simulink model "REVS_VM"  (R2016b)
settings: Solver=ode3  StartTime=REVS.sim_start_time_secs  StopTime=Inf  FixedStep=REVS.sim_step_time_secs  MaxStep=REVS.sim_step_time_secs  EnableMultiTasking=on
StopFcn:
  | postproc_datalog;
  | postproc_audit;
  | postproc_result;
model workspace (MATLAB code in the model file):
  other statements: REVS_setup_variants
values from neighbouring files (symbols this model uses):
  accessory = class_accessory_data    [class_test_data.m]
  battery = class_battery_data    [class_accessory_data.m]    (also in class_REVS_electric.m = class_REVS_battery)
  brake = struct(	'max_torque_Nm',[], 						'proportion_norm',1.0, 						'inertia_kgm2',0.0)    [class_REVS_drive_axle.m]
  engine = class_engine_data    [class_test_data.m]
  final_drive = struct(	'gear_ratio',[], 								'efficiency_norm',[], 								'inertia_kgm2',[] )    [class_REVS_drive_axle.m]
  gear = class_REVS_gearbox    [class_REVS_AT_transmission.m]
  tire = struct(	'radius_m',[], 						'rolling_resistance_coefficient',0, 						'vehicle_weight_norm',1.0,  						'wheel_slip_torque_Nm',[],  						'inertia_kgm2',0.0)    [class_REVS_drive_axle.m]
  torque_converter = class_REVS_torque_converter    [class_REVS_AT_transmission.m]
  transmission = class_transmission_data    [class_test_data.m]
  vehicle = class_vehicle_data    [class_test_data.m]
undefined symbols (not defined in the file or in its folder): alternator, ambient, controls, convert, DelayTimeSecs, drive_cycle, driver, electric, gear_strategy, InitialCondition, InitialValue, LoadSource, LookupStructure, MultiplyPosInputs, Normalize, NumPhases, REVS, SpeedSource, starter, tableshift, UpperSaturationLimit, Value, VerboseLevel, VerboseSignal
libraries: simulink x153
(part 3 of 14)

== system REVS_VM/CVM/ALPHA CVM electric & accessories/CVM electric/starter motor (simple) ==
  system_bus : Inport
  batt_volts_V : Inport  Port=2
  spd_in_radps : Inport  Port=3
  Bus Selector : BusSelector  OutputSignals=powertrain.control.ctrl_eng_on,powertrain.engine.ISC_state
  Divide1 : Product  Inputs=**//
  Divide2 : Product  Inputs=*/*
  Input Output Elec Mech E&P Nm radps V A : Subsystem
  PID Controller : simulink/Continuous/PID Controller  Controller=PID  TimeDomain=Continuous-time  SampleTime=-1  IntegratorMethod=Forward Euler  FilterMethod=Forward Euler  Form=Parallel  UseFilter=on  ControllerParametersSource=internal  P=10  I=10  D=0  N=1  InitialConditionSource=internal  InitialConditionForIntegrator=0  InitialConditionForFilter=0  ExternalReset=rising  ZeroCross=off  LimitOutput=on  UpperSaturationLimit=starter.max_torque_Nm  LowerSaturationLimit=0  LinearizeAsGain=on  AntiWindupMode=none  Kb=1  TrackingMode=off  Kt=1  PParamMin=[]  PParamMax=[]  IParamMin=[]  IParamMax=[]  DParamMin=[]  DParamMax=[]  NParamMin=[]  NParamMax=[]  KbParamMin=[]  KbParamMax=[]  KtParamMin=[]  KtParamMax=[]  POutMin=[]  POutMax=[]  IOutMin=[]  IOutMax=[]  DOutMin=[]  DOutMax=[]  NOutMin=[]  NOutMax=[]  KbOutMin=[]  KbOutMax=[]  KtOutMin=[]  KtOutMax=[]  IntegratorOutMin=[]  IntegratorOutMax=[]  FilterOutMin=[]  FilterOutMax=[]  SumOutMin=[]  SumOutMax=[]  SumI1OutMin=[]  SumI1OutMax=[]  SumI2OutMin=[]  SumI2OutMax=[]  SumI3OutMin=[]  SumI3OutMax=[]  SumDOutMin=[]  SumDOutMax=[]  SaturationOutMin=[]  SaturationOutMax=[]  IntegratorContinuousStateAttributes=''  IntegratorStateMustResolveToSignalObject=off  IntegratorRTWStateStorageClass=Auto  FilterContinuousStateAttributes=''  FilterStateMustResolveToSignalObject=off  FilterRTWStateStorageClass=Auto  DifferentiatorICPrevScaledInput=0  DifferentiatorOutMin=[]  DifferentiatorOutMax=[]
  Product : Product
  Rate Limiter : RateLimiter  RisingSlewLimit=electric.starter.max_torque_Nm * 10  FallingSlewLimit=-Inf
  Saturation1 : Saturate  UpperLimit=Inf  LowerLimit=eps
  Sum2 : Sum  Inputs=+-|
  cranking_speed_radps : Constant  Value=starter.cranking_speed_radps
  efficiency_norm : Constant  Value=starter.efficiency_norm
  efficiency_norm1 : Constant  Value=starter.rated_voltage_V
  inertia kgm2 : Constant  Value=starter.inertia_kgm2
  starter control : Subsystem
  to datalog1 : Subsystem
  to datalog2 : Subsystem
  to datalog3 : Subsystem
  trq_out_Nm : Outport
  iner_out_kgm2 : Outport  Port=2
  curr_out_A : Outport  Port=3
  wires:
  efficiency_norm1/1 -> Divide2/2
  Product/1 -> Divide2/1
  Divide1/1 -> Input Output Elec Mech E&P Nm radps V A/2(curr_in_A), curr_out_A/1
  Bus Selector/1 -> starter control/1(eng_on)  "<ctrl_eng_on>"
  system_bus/1 -> Bus Selector/1
  starter control/1(state) -> PID Controller/2, to datalog2/1(Var), Product/2
  PID Controller/1 -> Product/1, to datalog1/1(Var)
  Sum2/1 -> PID Controller/1
  cranking_speed_radps/1 -> Sum2/1
  Saturation1/1 -> Divide1/4
  efficiency_norm/1 -> Divide1/3
  batt_volts_V/1 -> Divide2/3, Input Output Elec Mech E&P Nm radps V A/1(volts_in_V), Saturation1/1, starter control/2(batt_volts_V)
  spd_in_radps/1 -> starter control/3(spd_in_radps), Sum2/2, Input Output Elec Mech E&P Nm radps V A/4(spd_out_radps), Divide1/2
  Divide2/1 -> to datalog3/1(Var), Rate Limiter/1
  inertia kgm2/1 -> iner_out_kgm2/1, Input Output Elec Mech E&P Nm radps V A/5(iner_out_kgm2)
  Rate Limiter/1 -> Input Output Elec Mech E&P Nm radps V A/3(trq_out_Nm), Divide1/1, trq_out_Nm/1
  Bus Selector/2 -> starter control/4(ISC_state)  "<ISC_state>"

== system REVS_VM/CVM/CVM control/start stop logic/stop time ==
  bool : Inport
  Constant : Constant  Value=Normalize
  Data Type Conversion2 : DataTypeConversion  OutDataTypeStr=double
  Integrator1 : Integrator  ExternalReset=falling  LimitOutput=on  UpperSaturationLimit=UpperSaturationLimit  LowerSaturationLimit=0
  Switch : Switch  Criteria=u2 > Threshold
  normalize : Gain  Gain=1/UpperSaturationLimit
  out : Outport
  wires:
  Switch/1 -> out/1
  normalize/1 -> Switch/1
  Integrator1/1 -> Switch/3, normalize/1
  Constant/1 -> Switch/2
  bool/1 -> Data Type Conversion2/1
  Data Type Conversion2/1 -> Integrator1/1, Integrator1/2

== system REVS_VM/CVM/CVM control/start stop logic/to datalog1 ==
  Var : Inport
  Constant : Constant  Value=VerboseSignal
  Constant1 : Constant  Value=VerboseLevel
  Relational Operator : RelationalOperator  OutDataTypeStr=boolean  ZeroCross=off
  Subsystem : Subsystem
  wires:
  Constant1/1 -> Relational Operator/2
  Constant/1 -> Relational Operator/1
  Relational Operator/1 -> Subsystem/Enable
  Var/1 -> Subsystem/1(In1)

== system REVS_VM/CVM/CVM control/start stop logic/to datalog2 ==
  Var : Inport
  Constant : Constant  Value=VerboseSignal
  Constant1 : Constant  Value=VerboseLevel
  Relational Operator : RelationalOperator  OutDataTypeStr=boolean  ZeroCross=off
  Subsystem : Subsystem
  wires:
  Constant1/1 -> Relational Operator/2
  Constant/1 -> Relational Operator/1
  Relational Operator/1 -> Subsystem/Enable
  Var/1 -> Subsystem/1(In1)

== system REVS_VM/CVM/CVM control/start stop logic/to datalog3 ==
  Var : Inport
  Constant : Constant  Value=VerboseSignal
  Constant1 : Constant  Value=VerboseLevel
  Relational Operator : RelationalOperator  OutDataTypeStr=boolean  ZeroCross=off
  Subsystem : Subsystem
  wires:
  Constant1/1 -> Relational Operator/2
  Constant/1 -> Relational Operator/1
  Relational Operator/1 -> Subsystem/Enable
  Var/1 -> Subsystem/1(In1)

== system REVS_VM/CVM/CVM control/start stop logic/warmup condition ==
  bus : Inport
  Bus Creator : BusCreator  Inputs=10
  Bus Creator1 : BusCreator  Inputs=2
  Bus Selector : BusSelector  OutputSignals=var_sigs.var_sig1  OutputAsBus=on
  Data Type Conversion : DataTypeConversion  OutDataTypeStr=double
  Display : Display
  Fcn : Fcn
  Variable {1..10} (10 alike) : Constant  Value=nan
  out : Outport
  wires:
  Data Type Conversion/1 -> Fcn/1
  Bus Selector/1 -> Data Type Conversion/1, Display/1
  Bus Creator1/1 -> Bus Selector/1
  Fcn/1 -> out/1
  bus/1 -> Bus Creator1/1  "system_bus"
  Bus Creator/1 -> Bus Creator1/2  "var_sigs"
  Variable 1/1 -> Bus Creator/1  "var_sig1"
  Variable 2/1 -> Bus Creator/2  "var_sig2"
  Variable 3/1 -> Bus Creator/3  "var_sig3"
  Variable 4/1 -> Bus Creator/4  "var_sig4"
  Variable 5/1 -> Bus Creator/5  "var_sig5"
  Variable 6/1 -> Bus Creator/6  "var_sig6"
  Variable 7/1 -> Bus Creator/7  "var_sig7"
  Variable 8/1 -> Bus Creator/8  "var_sig8"
  Variable 9/1 -> Bus Creator/9  "var_sig9"
  Variable 10/1 -> Bus Creator/10  "var_sig10"

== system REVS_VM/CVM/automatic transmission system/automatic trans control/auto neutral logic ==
  system_bus : Inport
  Bus Selector : BusSelector  OutputSignals=vehicle.veh_spd_mps,driver.accel_anticipate_bool,powertrain.control.ctrl_eng_on,powertrain.engine.eng_spd_radps
  Compare To Constant : simulink/Logic and Bit Operations/Compare To Constant  relop=>=  const=transmission.control.auto_neutral_delay_secs  OutDataTypeStr=boolean
  Compare To Zero4 : simulink/Logic and Bit Operations/Compare To Zero  relop=>  OutDataTypeStr=boolean
  Gain : Gain  Gain=1.5
  Logical Operator1 : Logic  Operator=OR  AllPortsSameDT=off  OutDataTypeStr=boolean
  Logical Operator2 : Logic  Inputs=4  AllPortsSameDT=off  OutDataTypeStr=boolean
  Logical Operator3 : Logic  Operator=NOT  AllPortsSameDT=off  OutDataTypeStr=boolean
  Logical Operator4 : Logic  Inputs=3  AllPortsSameDT=off  OutDataTypeStr=boolean
  Relational Operator : RelationalOperator  Operator=<  OutDataTypeStr=boolean
  auto neutral enable : Constant  Value=transmission.control.auto_neutral_enable
  crank speed : Constant  Value=electric.starter.cranking_speed_radps
  stop time : Subsystem
  stopped speed : simulink/Logic and Bit Operations/Compare To Constant  relop=<=  const=0.1  OutDataTypeStr=boolean
  to datalog1 : Subsystem
  warmup condition : Subsystem
  auto_neutral_bool : Outport
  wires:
  system_bus/1 -> warmup condition/1(bus), Bus Selector/1
  stop time/1(out) -> Compare To Constant/1
  stopped speed/1 -> stop time/1(bool), Logical Operator4/2
  warmup condition/1(out) -> Logical Operator2/4
  Compare To Zero4/1 -> Logical Operator3/1
  auto neutral enable/1 -> Logical Operator2/1
  Logical Operator3/1 -> Logical Operator2/3
  Bus Selector/1 -> stopped speed/1  "<veh_spd_mps>"
  Compare To Constant/1 -> Logical Operator2/2
  Logical Operator1/1 -> auto_neutral_bool/1, to datalog1/1(Var)
  Bus Selector/2 -> Compare To Zero4/1  "<accel_anticipate_bool>"
  Logical Operator4/1 -> Logical Operator1/2
  Logical Operator2/1 -> Logical Operator1/1
  Bus Selector/3 -> Logical Operator4/1  "<ctrl_eng_on>"
  Relational Operator/1 -> Logical Operator4/3
  Bus Selector/4 -> Relational Operator/1  "<eng_spd_radps>"
  crank speed/1 -> Gain/1
  Gain/1 -> Relational Operator/2

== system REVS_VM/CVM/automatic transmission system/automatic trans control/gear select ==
  note: 1) Only subsystems can be added as variant choices at this level 2) Blocks cannot be connected at this level as connectivity is automatically determined at simulation, based on the active variant
  system_bus : Inport
  ALPHAshift : Subsystem  VariantControl=get_REVS_transmission_gear_strategy_type(transmission) == enum_transmission_gear_select.ALPHAshift
  ALPHAshift_CVT : Subsystem  VariantControl=get_REVS_transmission_gear_strategy_type(transmission) == enum_transmission_gear_select.ALPHAshift_CVT
  SUBARUshift_CVT : Subsystem  VariantControl=get_REVS_transmission_gear_strategy_type(transmission) == enum_transmission_gear_select.subarushift_CVT
  autoshift 3 : Subsystem  VariantControl=get_REVS_transmission_gear_strategy_type(transmission) == enum_transmission_gear_select.autoshift3
  external gear select : Subsystem  VariantControl=get_REVS_transmission_gear_strategy_type(transmission) == enum_transmission_gear_select.externalshift
  external ratio select CVT : Subsystem  VariantControl=get_REVS_transmission_gear_strategy_type(transmission) == enum_transmission_gear_select.externalshift_CVT
  table gear select : Subsystem  VariantControl=get_REVS_transmission_gear_strategy_type(transmission) == enum_transmission_gear_select.tableshift
  table gear select with skip shift : Subsystem  VariantControl=get_REVS_transmission_gear_strategy_type(transmission) == enum_transmission_gear_select.tableshift_skipshift
  target_gear : Outport

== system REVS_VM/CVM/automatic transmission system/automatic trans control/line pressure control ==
  system_bus : Inport
  Rate Limiter : RateLimiter  RisingSlewLimit=transmission.control.line_press_rate_limit_barps  FallingSlewLimit=-Inf  InitialCondition=3
  dynamic lookup : Subsystem
  cmd_line_press_bar : Outport
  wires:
  system_bus/1 -> dynamic lookup/1(bus)
  dynamic lookup/1(out) -> Rate Limiter/1
  Rate Limiter/1 -> cmd_line_press_bar/1

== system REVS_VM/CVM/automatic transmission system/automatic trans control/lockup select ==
  note: 1) Only subsystems can be added as variant choices at this level 2) Blocks cannot be connected at this level as connectivity is automatically determined at simulation, based on the active variant
  gear_number : Inport
  system_bus : Inport  Port=2
  3-state lockup rules uber : Subsystem  VariantControl="get_REVS_transmission_tcc_strategy_type(transmission)  == enum_transmission_lockup_select.uber_dynamic_3state"
  "external lockup " : Subsystem  VariantControl="get_REVS_transmission_tcc_strategy_type(transmission)  == enum_transmission_lockup_select.external_lockup"
  lockup rules dynamic expression : Subsystem  VariantControl="get_REVS_transmission_tcc_strategy_type(transmission)  == enum_transmission_lockup_select.lockup_rules_dynamic_expression"
  lockup rules speed select : Subsystem  VariantControl="get_REVS_transmission_tcc_strategy_type(transmission)  == enum_transmission_lockup_select.lockup_rules_speed_select"
  lockup rules uber : Subsystem  VariantControl="get_REVS_transmission_tcc_strategy_type(transmission)  == enum_transmission_lockup_select.uber_dynamic"
  table lockup : Subsystem  VariantControl="get_REVS_transmission_tcc_strategy_type(transmission)  == enum_transmission_lockup_select.table_lockup"
  lockup_cmd : Outport

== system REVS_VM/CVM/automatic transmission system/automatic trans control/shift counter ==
  target_gear : Inport
  Constant : Constant  Value=transmission.gear.number
  Last Gear : Memory  X0=1
  Memory : Memory  X0=1
  Relational Operator : RelationalOperator  Operator===  OutDataTypeStr=boolean  ZeroCross=off
  Relational Operator1 : RelationalOperator  Operator=>  OutDataTypeStr=boolean  ZeroCross=off
  Relational Operator2 : RelationalOperator  Operator=<  OutDataTypeStr=boolean  ZeroCross=off
  Reshape : Reshape
  Switch : Switch  Criteria=u2 > Threshold
  downshifft result counter : Subsystem
  result integrator : Subsystem
  uppshift result counter : Subsystem
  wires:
  Relational Operator2/1 -> downshifft result counter/1(in)
  Last Gear/1 -> Relational Operator1/2, Relational Operator2/2
  Memory/1 -> Switch/3
  Switch/1 -> Memory/1, Relational Operator1/1, Relational Operator2/1, Last Gear/1
  target_gear/1 -> Switch/2, Switch/1, Relational Operator/1
  Reshape/1 -> Relational Operator/2
  Relational Operator/1 -> result integrator/1(in)
  Constant/1 -> Reshape/1
  Relational Operator1/1 -> uppshift result counter/1(in)

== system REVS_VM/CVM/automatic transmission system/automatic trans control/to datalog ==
  Var : Inport
  Constant : Constant  Value=VerboseSignal
  Constant1 : Constant  Value=VerboseLevel
  Relational Operator : RelationalOperator  OutDataTypeStr=boolean  ZeroCross=off
  Subsystem : Subsystem
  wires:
  Constant1/1 -> Relational Operator/2
  Constant/1 -> Relational Operator/1
  Relational Operator/1 -> Subsystem/Enable
  Var/1 -> Subsystem/1(In1)

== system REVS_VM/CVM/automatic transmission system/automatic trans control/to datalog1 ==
  Var : Inport
  Constant : Constant  Value=VerboseSignal
  Constant1 : Constant  Value=VerboseLevel
  Relational Operator : RelationalOperator  OutDataTypeStr=boolean  ZeroCross=off
  Subsystem : Subsystem
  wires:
  Constant1/1 -> Relational Operator/2
  Constant/1 -> Relational Operator/1
  Relational Operator/1 -> Subsystem/Enable
  Var/1 -> Subsystem/1(In1)

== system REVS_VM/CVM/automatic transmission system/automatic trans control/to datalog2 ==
  Var : Inport
  Constant : Constant  Value=VerboseSignal
  Constant1 : Constant  Value=VerboseLevel
  Relational Operator : RelationalOperator  OutDataTypeStr=boolean  ZeroCross=off
  Subsystem : Subsystem
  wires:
  Constant1/1 -> Relational Operator/2
  Constant/1 -> Relational Operator/1
  Relational Operator/1 -> Subsystem/Enable
  Var/1 -> Subsystem/1(In1)

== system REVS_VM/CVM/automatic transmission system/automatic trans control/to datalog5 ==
  Var : Inport
  Constant : Constant  Value=VerboseSignal
  Constant1 : Constant  Value=VerboseLevel
  Relational Operator : RelationalOperator  OutDataTypeStr=boolean  ZeroCross=off
  Subsystem : Subsystem
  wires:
  Constant1/1 -> Relational Operator/2
  Constant/1 -> Relational Operator/1
  Relational Operator/1 -> Subsystem/Enable
  Var/1 -> Subsystem/1(In1)

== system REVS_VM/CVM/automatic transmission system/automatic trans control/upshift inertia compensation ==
  system_bus : Inport
  Bus Selector : BusSelector  OutputSignals=powertrain.trans.ctrl.gear_num,powertrain.trans.core.gearbox.gb_curr_gear,powertrain.trans.ctrl.tcc_lockup_cmd_bool,powertrain.trans.trq_conv.tcc_lockup_bool
  Logical Operator : Logic  Operator=OR  AllPortsSameDT=off  OutDataTypeStr=boolean
  Logical Operator1 : Logic  AllPortsSameDT=off  OutDataTypeStr=boolean
  Relational Operator : RelationalOperator  Operator=>  OutDataTypeStr=boolean
  Relational Operator1 : RelationalOperator  Operator=>  OutDataTypeStr=boolean
  comp_iner_enable : Outport
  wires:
  Logical Operator1/1 -> Logical Operator/1
  Relational Operator/1 -> Logical Operator1/1
  system_bus/1 -> Bus Selector/1
  Relational Operator1/1 -> Logical Operator/2
  Bus Selector/4 -> Relational Operator1/2, Logical Operator1/2  "<tcc_lockup_bool>"
  Bus Selector/3 -> Relational Operator1/1  "<tcc_lockup_cmd_bool>"
  Logical Operator/1 -> comp_iner_enable/1  "eng_comp_iner_enable"
  Bus Selector/1 -> Relational Operator/1  "<gear_num>"
  Bus Selector/2 -> Relational Operator/2  "<gb_curr_gear>"

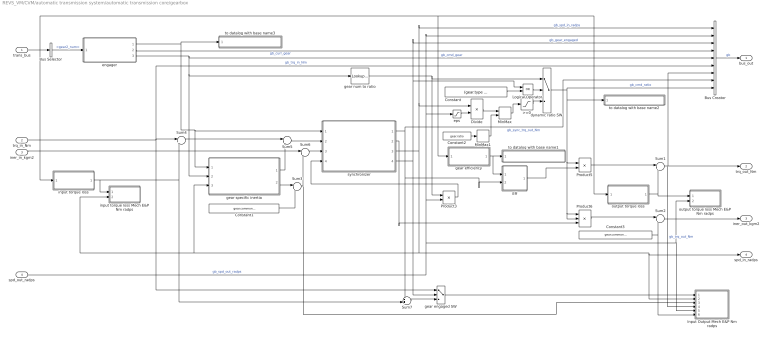
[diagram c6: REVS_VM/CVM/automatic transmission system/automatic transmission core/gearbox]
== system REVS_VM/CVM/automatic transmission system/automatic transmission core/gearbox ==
  trans_bus : Inport
  trq_in_Nm : Inport  Port=2
  iner_in_kgm2 : Inport  Port=3
  spd_out_radps : Inport  Port=4
  >=0 : Saturate  UpperLimit=Inf  LowerLimit=0
  Bus Creator : BusCreator  Inputs=9
  Bus Selector : BusSelector  OutputSignals=gear_num
  Constant : Constant  Value=(gear.type == enum_transmission_type.AMT) || (gear.type == enum_transmission_type.manual) || (gear.type == enum_transmission_type.DCT)
  Constant1 : Constant  Value=gear.common_input_inertia_kgm2
  Constant2 : Constant  Value=gear.ratio
  Constant3 : Constant  Value=gear.common_output_inertia_kgm2
  Divide : Product  Inputs=*/
  Eff : Subsystem
  Input Output Mech E&P Nm radps : Subsystem
  Logical Operator : Logic  Operator=OR  AllPortsSameDT=off  OutDataTypeStr=boolean
  MinMax : MinMax  Inputs=2
  MinMax1 : MinMax  Function=max
  Product3 : Product
  Product5 : Product
  Product6 : Product  Inputs=3
  Sum1 : Sum  Inputs=|+-
  Sum2 : Sum  Inputs=|++
  Sum3 : Sum  Inputs=|++
  Sum4 : Sum  Inputs=|+-
  Sum5 : Sum  Inputs=|+-
  Sum6 : Sum  Inputs=|++
  Sum7 : Sum  Inputs=++|
  dynamic ratio SW : Switch  Threshold=1
  engager : Subsystem
  eps : Saturate  UpperLimit=Inf  LowerLimit=1
  gear efficiency : Subsystem
  gear engaged SW : Switch  Threshold=1
  gear num to ratio : Lookup_n-D  NumberOfTableDimensions=1  BreakpointsForDimension1=gear.number  IndexSearchMethod=Linear search  BeginIndexSearchUsingPreviousIndexResult=on  Table=gear.ratio  ExtrapMethod=Clip  DiagnosticForOutOfRangeInput=Error  InternalRulePriority=Speed  RndMeth=Simplest
  gear specific inertia : Subsystem
  input torque loss : Subsystem
  input torque loss Mech E&P Nm radps : Subsystem
  output torque loss : Subsystem
  output torque loss Mech E&P Nm radps : Subsystem
  synchronizer : Subsystem
  to datalog with base name1 : Subsystem
  to datalog with base name2 : Subsystem
  to datalog with base name3 : Subsystem
  bus_out : Outport
  trq_out_Nm : Outport  Port=2
  iner_out_kgm2 : Outport  Port=3
  spd_in_radps : Outport  Port=4
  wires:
  MinMax/1 -> >=0/1
  >=0/1 -> dynamic ratio SW/3
  MinMax1/1 -> MinMax/2
  Constant2/1 -> MinMax1/1
  Divide/1 -> MinMax/1
  Product5/1 -> Sum1/1
  output torque loss/1(out) -> output torque loss Mech E&P Nm radps/1(trq_Nm), Sum1/2
  spd_out_radps/1 -> output torque loss Mech E&P Nm radps/2(spd_radps), Input Output Mech E&P Nm radps/5(spd_out_radps), Bus Creator/2, eps/1, Product3/2  "gb_spd_out_radps"
  trans_bus/1 -> output torque loss/1(bus), gear efficiency/1(bus), input torque loss/1(bus), Bus Selector/1
  Constant/1 -> Logical Operator/2
  Logical Operator/1 -> dynamic ratio SW/2
  dynamic ratio SW/1 -> Product5/1, Product6/1, Product6/2, to datalog with base name2/1(Var), Bus Creator/9  "gb_cmd_ratio"
  eps/1 -> Divide/2
  gear engaged SW/1 -> Input Output Mech E&P Nm radps/1(trq_in_Nm)
  Product3/1 -> synchronizer/4(sync_spd_out_radps)
  input torque loss/1(out) -> input torque loss Mech E&P Nm radps/1(trq_Nm), Sum7/2, Sum4/2
  Bus Selector/1 -> engager/1(tgt_gear_num)  "<gear2_num>"
  engager/3(cmd_gear_num) -> Bus Creator/5, gear specific inertia/2(cmd_gear_num), gear num to ratio/1  "gb_cmd_gear"
  Sum6/1 -> synchronizer/3(sync_iner_in_kgm2)
  Sum4/1 -> Sum5/1
  Constant3/1 -> Input Output Mech E&P Nm radps/6(iner_out_kgm2), Sum2/2
  Product6/1 -> Sum2/1
  iner_in_kgm2/1 -> Sum6/1
  Sum1/1 -> Bus Creator/7, trq_out_Nm/1, Input Output Mech E&P Nm radps/4(trq_out_Nm)  "gb_trq_out_Nm"
  synchronizer/3(sync_spd_in_radps) -> Bus Creator/1, Divide/1, gear specific inertia/3(iner_spd_out_radps), input torque loss Mech E&P Nm radps/2(spd_radps), spd_in_radps/1, Input Output Mech E&P Nm radps/2(spd_in_radps)  "gb_spd_in_radps"
  Bus Creator/1 -> bus_out/1  "gb"
  gear efficiency/1(out) -> to datalog with base name1/1(Var), Eff/1(Efficiency)
  Eff/1(Output) -> Product5/2
  synchronizer/1(sync_trq_out_Nm) -> Sum7/1, Eff/2(Input), Bus Creator/8  "gb_sync_trq_out_Nm"
  synchronizer/2(sync_iner_out_kgm2) -> Product6/3
  engager/1(engage) -> gear specific inertia/1(engage), synchronizer/1(engage), to datalog with base name3/1(Var)
  Sum2/1 -> iner_out_kgm2/1
  Constant1/1 -> Sum3/2
  trq_in_Nm/1 -> Sum4/1, Bus Creator/6, gear engaged SW/1  "gb_trq_in_Nm"
  Sum5/1 -> synchronizer/2(sync_trq_in_Nm)
  gear specific inertia/1(iner_trq_out_Nm) -> Sum5/2
  Sum3/1 -> Input Output Mech E&P Nm radps/3(iner_in_kgm2), Sum6/2
  synchronizer/4(sync_lockup) -> gear engaged SW/2, Bus Creator/3, Logical Operator/1  "gb_gear_engaged"
  Sum7/1 -> gear engaged SW/3
  gear specific inertia/2(iner_out_kgm2) -> Sum3/1
  gear num to ratio/1 -> dynamic ratio SW/1, Product3/1
  engager/2(curr_gear_num) -> Bus Creator/4  "gb_curr_gear"

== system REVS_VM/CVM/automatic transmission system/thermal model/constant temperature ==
  system_bus : Inport
  Bus Creator : BusCreator  Inputs=1
  Constant : Constant  Value=transmission.thermal.temperature_degC
  thermal_bus : Outport
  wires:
  Bus Creator/1 -> thermal_bus/1
  Constant/1 -> Bus Creator/1  "trans_temp_degC"

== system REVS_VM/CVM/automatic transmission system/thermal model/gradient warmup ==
  system_bus : Inport
  Bus Creator : BusCreator  Inputs=1
  Constant : Constant  Value=transmission.thermal.final_temperature_degC
  State-Space : StateSpace  A=-1/transmission.thermal.gradient_time_constant_sec  C=1/transmission.thermal.gradient_time_constant_sec  D=0  X0=transmission.thermal.initial_temperature_degC  ContinuousStateAttributes='temperature'
  thermal_bus : Outport
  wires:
  Constant/1 -> State-Space/1
  Bus Creator/1 -> thermal_bus/1
  State-Space/1 -> Bus Creator/1  "trans_temp_degC"

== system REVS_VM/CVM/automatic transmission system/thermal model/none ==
  system_bus : Inport
  thermal_bus : Outport

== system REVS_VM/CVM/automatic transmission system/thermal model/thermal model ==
  system_bus : Inport
  Bus Creator : BusCreator  Inputs=1
  Constant : Constant  Value=0
  Constant1 : Constant  Value=transmission.thermal.initial_temperature_degC
  Constant2 : Constant  Value=transmission.thermal.capacity_JpK
  Constant4 : Constant  Value=transmission.thermal.target_temperature_degC
  Constant5 : Constant  Value=transmission.thermal.passive_conductance_WpK
  Constant6 : Constant  Value=transmission.thermal.cooling_conductance_WpK
  Integrator1 : Integrator  ExternalReset=level  InitialConditionSource=external  InitialCondition=transmission.thermal.initial_temperature_degC  ZeroCross=off
  MinMax : MinMax  Function=max  Inputs=2
  Product3 : Product  Inputs=**
  Product4 : Product  Inputs=***
  Product5 : Product  Inputs=*/
  RelayCooling : Relay  OnSwitchValue=1  OffSwitchValue=-1  ZeroCross=off
  Saturation : Saturate  UpperLimit=Inf  LowerLimit=eps
  Step : Step  Before=1  After=0  SampleTime=0  ZeroCross=off
  Subtract2 : Sum  Inputs=+-
  Subtract3 : Sum  Inputs=+-
  Sum of Elements : Sum  Inputs=+
  Sum of Elements1 : Sum  Inputs=+
  Sum3 : Sum  Inputs=+--
  conduction temperatures : Subsystem
  lowpass filter : TransferFcn  Denominator=[1 1]
  power loss signals : Subsystem
  to datalog1 : Subsystem
  to datalog2 : Subsystem
  to datalog3 : Subsystem
  to datalog4 : Subsystem
  to datalog5 : Subsystem
  to datalog6 : Subsystem
  thermal_bus : Outport
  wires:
  Step/1 -> Integrator1/2
  Constant1/1 -> Integrator1/3
  Subtract2/1 -> RelayCooling/1
  RelayCooling/1 -> Product4/1  "temp_ctrl_state"
  Constant4/1 -> Subtract2/2
  Bus Creator/1 -> thermal_bus/1
  MinMax/1 -> lowpass filter/1
  Saturation/1 -> Product5/2
  Constant2/1 -> Saturation/1
  Integrator1/1 -> to datalog1/1(Var), Subtract3/1, Subtract2/1, Bus Creator/1  "trans_temp_degC"
  Sum3/1 -> to datalog3/1(Var), Product5/1
  Product5/1 -> Integrator1/1
  lowpass filter/1 -> to datalog2/1(Var), Sum3/1
  system_bus/1 -> power loss signals/1(bus), conduction temperatures/1(bus)
  power loss signals/1(out) -> MinMax/2
  Constant/1 -> MinMax/1
  conduction temperatures/1(out) -> to datalog6/1(Var), Subtract3/2
  Subtract3/1 -> Product4/3, Product3/2
  Constant5/1 -> Product3/1
  Constant6/1 -> Product4/2
  Sum of Elements1/1 -> Sum3/3
  Sum of Elements/1 -> Sum3/2
  Product3/1 -> to datalog4/1(Var), Sum of Elements1/1
  Product4/1 -> to datalog5/1(Var), Sum of Elements/1

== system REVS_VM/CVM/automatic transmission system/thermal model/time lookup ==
  system_bus : Inport
  1-D Lookup Table : Lookup_n-D  NumberOfTableDimensions=1  BreakpointsForDimension1=transmission.thermal.temperature_time_sec  IndexSearchMethod=Linear search  BeginIndexSearchUsingPreviousIndexResult=on  Table=transmission.thermal.temperature_degC  ExtrapMethod=Clip  InternalRulePriority=Speed  RndMeth=Simplest
  Bus Creator : BusCreator  Inputs=1
  Bus Selector : BusSelector  OutputSignals=driver.cycle_pos_secs
  thermal_bus : Outport
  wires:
  system_bus/1 -> Bus Selector/1
  Bus Creator/1 -> thermal_bus/1
  1-D Lookup Table/1 -> Bus Creator/1  "trans_temp_degC"
  Bus Selector/1 -> 1-D Lookup Table/1  "<cycle_pos_secs>"

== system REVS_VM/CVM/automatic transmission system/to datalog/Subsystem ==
  In1 : Inport
  Enable : EnablePort
  To Workspace : ToWorkspace  VariableName=datalog__transmission__output_torque_Nm  SampleTime=-1
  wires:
  In1/1 -> To Workspace/1

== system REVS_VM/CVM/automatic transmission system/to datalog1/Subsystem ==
  In1 : Inport
  Enable : EnablePort
  To Workspace : ToWorkspace  VariableName=datalog__transmission__output_inertia_kgm2  SampleTime=-1
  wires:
  In1/1 -> To Workspace/1

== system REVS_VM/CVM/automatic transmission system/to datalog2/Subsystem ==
  In1 : Inport
  Enable : EnablePort
  To Workspace : ToWorkspace  VariableName=datalog__transmission__output_speed_radps  SampleTime=-1
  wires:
  In1/1 -> To Workspace/1

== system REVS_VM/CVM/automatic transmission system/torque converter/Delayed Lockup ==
  Engage : Inport
  Compare To Constant : simulink/Logic and Bit Operations/Compare To Constant  relop=>  const=0.9  OutDataTypeStr=boolean
  Compare To Constant1 : simulink/Logic and Bit Operations/Compare To Constant  relop=>=  const=1  OutDataTypeStr=boolean
  Logical Operator2 : Logic  AllPortsSameDT=off  OutDataTypeStr=boolean
  Memory1 : Memory
  Lockup : Outport
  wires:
  Logical Operator2/1 -> Lockup/1
  Memory1/1 -> Logical Operator2/1
  Engage/1 -> Compare To Constant/1, Compare To Constant1/1
  Compare To Constant/1 -> Logical Operator2/2
  Compare To Constant1/1 -> Memory1/1

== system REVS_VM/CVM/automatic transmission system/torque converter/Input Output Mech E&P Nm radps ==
  trq_in_Nm : Inport
  spd_in_radps : Inport  Port=2
  iner_in_kgm2 : Inport  Port=3
  trq_out_Nm : Inport  Port=4
  spd_out_radps : Inport  Port=5
  iner_out_kgm2 : Inport  Port=6
  Compare To Constant : simulink/Logic and Bit Operations/Compare To Constant  relop=>=  const=1  OutDataTypeStr=boolean
  Constant : Constant  Value=VerboseSignal
  Subsystem : Subsystem
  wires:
  trq_in_Nm/1 -> Subsystem/1(trq_in_Nm)
  spd_in_radps/1 -> Subsystem/2(spd_in_radps)
  iner_in_kgm2/1 -> Subsystem/3(iner_in_kgm2)
  trq_out_Nm/1 -> Subsystem/4(trq_out_Nm)
  spd_out_radps/1 -> Subsystem/5(spd_out_radps)
  iner_out_kgm2/1 -> Subsystem/6(iner_out_kgm2)
  Compare To Constant/1 -> Subsystem/Enable
  Constant/1 -> Compare To Constant/1

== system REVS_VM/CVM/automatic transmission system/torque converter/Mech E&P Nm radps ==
  trq_Nm : Inport
  spd_radps : Inport  Port=2
  Compare To Constant : simulink/Logic and Bit Operations/Compare To Constant  relop=>=  const=1  OutDataTypeStr=boolean
  Constant : Constant  Value=VerboseSignal
  Subsystem : Subsystem
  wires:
  trq_Nm/1 -> Subsystem/1(trq_Nm)
  spd_radps/1 -> Subsystem/2(spd_radps)
  Compare To Constant/1 -> Subsystem/Enable
  Constant/1 -> Compare To Constant/1

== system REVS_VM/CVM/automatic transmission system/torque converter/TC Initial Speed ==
  In : Inport
  Constant2 : Constant
  IC Switch : Switch  Criteria=u2 ~= 0
  IC Value : Constant  Value=InitialValue
  Memory : Memory
  Out : Outport
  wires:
  Constant2/1 -> Memory/1
  Memory/1 -> IC Switch/2
  IC Value/1 -> IC Switch/3
  In/1 -> IC Switch/1
  IC Switch/1 -> Out/1

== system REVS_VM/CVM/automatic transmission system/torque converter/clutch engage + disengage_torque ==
  engage : Inport
  trq_in_Nm : Inport  Port=2
  final_spd_radps : Inport  Port=3
  current_spd_radps : Inport  Port=4
  iner_in_kgm2 : Inport  Port=5
  Detect Increase : simulink/Logic and Bit Operations/Detect Increase  vinit=0.0  InputProcessing=Inherited  OutDataTypeStr=boolean
  Product1 : Product
  Sum : Sum  Inputs=+-|
  engage target speed calc : Subsystem
  engage trq : Product  Inputs=3
  tcc_torque_Nm : Outport
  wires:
  current_spd_radps/1 -> engage target speed calc/3(current_spd_radps)
  final_spd_radps/1 -> engage target speed calc/2(final_spd_radps)
  engage/1 -> engage target speed calc/1(engage), Detect Increase/1, Product1/1
  trq_in_Nm/1 -> Product1/2
  Product1/1 -> Sum/1
  iner_in_kgm2/1 -> engage trq/3
  Sum/1 -> tcc_torque_Nm/1
  engage trq/1 -> Sum/2
  Detect Increase/1 -> engage trq/1
  engage target speed calc/1(engage_accel_radps2) -> engage trq/2

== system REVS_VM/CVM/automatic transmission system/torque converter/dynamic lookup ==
  bus : Inport
  Bus Selector : BusSelector  OutputSignals=gb.gb_cmd_gear,gb_spd_in_radps,ctrl.gb_line_press_bar
  Lookup : Lookup_n-D  NumberOfTableDimensions=10  BreakpointsForDimension1=LookupStructure.axis_1.breakpoints  BreakpointsForDimension2=LookupStructure.axis_2.breakpoints  BreakpointsForDimension3=LookupStructure.axis_3.breakpoints  BreakpointsForDimension4=LookupStructure.axis_4.breakpoints  BreakpointsForDimension5=LookupStructure.axis_5.breakpoints  BreakpointsForDimension6=LookupStructure.axis_6.breakpoints  BreakpointsForDimension7=LookupStructure.axis_7.breakpoints  BreakpointsForDimension8=LookupStructure.axis_8.breakpoints  BreakpointsForDimension9=LookupStructure.axis_9.breakpoints  BreakpointsForDimension10=LookupStructure.axis_10.breakpoints  IndexSearchMethod=Linear search  BeginIndexSearchUsingPreviousIndexResult=on  Table=LookupStructure.table  DiagnosticForOutOfRangeInput=Warning  InternalRulePriority=Speed  RndMeth=Simplest  SupportTunableTableSize=on  MaximumIndicesForEachDimension=LookupStructure.table_size
  out : Outport
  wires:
  bus/1 -> Bus Selector/1
  Lookup/1 -> out/1

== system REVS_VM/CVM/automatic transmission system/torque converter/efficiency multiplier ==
  efficiency : Inport
  input : Inport  Port=2
  Constant4 : Constant  Value=MultiplyPosInputs
  Math Function : Math  Operator=reciprocal
  Math Function1 : Math  Operator=reciprocal
  Product1 : Product
  Product2 : Product
  Switch : Switch  ZeroCross=off
  Switch1 : Switch  ZeroCross=off
  Switch2 : Switch  Criteria=u2 > Threshold  ZeroCross=off
  output : Outport
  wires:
  Constant4/1 -> Switch2/2
  Product2/1 -> Switch2/3
  Product1/1 -> Switch2/1
  Switch2/1 -> output/1
  Math Function1/1 -> Switch1/1
  input/1 -> Switch1/2, Product2/1, Product1/2, Switch/2
  efficiency/1 -> Switch/1, Math Function/1, Math Function1/1, Switch1/3
  Switch1/1 -> Product2/2
  Math Function/1 -> Switch/3
  Switch/1 -> Product1/1

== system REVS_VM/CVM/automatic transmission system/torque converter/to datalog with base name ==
  Var : Inport
  Constant : Constant  Value=VerboseSignal
  Constant1 : Constant  Value=VerboseLevel
  Relational Operator : RelationalOperator  OutDataTypeStr=boolean  ZeroCross=off
  Subsystem : Subsystem
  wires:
  Constant1/1 -> Relational Operator/2
  Relational Operator/1 -> Subsystem/Enable
  Constant/1 -> Relational Operator/1
  Var/1 -> Subsystem/1(Var)

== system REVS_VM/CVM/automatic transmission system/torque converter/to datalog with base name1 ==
  Var : Inport
  Constant : Constant  Value=VerboseSignal
  Constant1 : Constant  Value=VerboseLevel
  Relational Operator : RelationalOperator  OutDataTypeStr=boolean  ZeroCross=off
  Subsystem : Subsystem
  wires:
  Constant1/1 -> Relational Operator/2
  Relational Operator/1 -> Subsystem/Enable
  Constant/1 -> Relational Operator/1
  Var/1 -> Subsystem/1(Var)

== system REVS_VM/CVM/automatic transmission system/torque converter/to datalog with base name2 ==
  Var : Inport
  Constant : Constant  Value=VerboseSignal
  Constant1 : Constant  Value=VerboseLevel
  Relational Operator : RelationalOperator  OutDataTypeStr=boolean  ZeroCross=off
  Subsystem : Subsystem
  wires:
  Constant1/1 -> Relational Operator/2
  Relational Operator/1 -> Subsystem/Enable
  Constant/1 -> Relational Operator/1
  Var/1 -> Subsystem/1(Var)

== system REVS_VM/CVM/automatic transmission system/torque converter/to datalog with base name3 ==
  Var : Inport
  Constant : Constant  Value=VerboseSignal
  Constant1 : Constant  Value=VerboseLevel
  Relational Operator : RelationalOperator  OutDataTypeStr=boolean  ZeroCross=off
  Subsystem : Subsystem
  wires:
  Constant1/1 -> Relational Operator/2
  Relational Operator/1 -> Subsystem/Enable
  Constant/1 -> Relational Operator/1
  Var/1 -> Subsystem/1(Var)

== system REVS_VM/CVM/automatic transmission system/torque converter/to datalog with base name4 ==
  Var : Inport
  Constant : Constant  Value=VerboseSignal
  Constant1 : Constant  Value=VerboseLevel
  Relational Operator : RelationalOperator  OutDataTypeStr=boolean  ZeroCross=off
  Subsystem : Subsystem
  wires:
  Constant1/1 -> Relational Operator/2
  Relational Operator/1 -> Subsystem/Enable
  Constant/1 -> Relational Operator/1
  Var/1 -> Subsystem/1(Var)

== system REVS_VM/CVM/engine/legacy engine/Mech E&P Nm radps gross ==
  " trq_Nm" : Inport
  spd_radps : Inport  Port=2
  iner_kgm2 : Inport  Port=3
  Compare To Constant : simulink/Logic and Bit Operations/Compare To Constant  relop=>=  const=1  OutDataTypeStr=boolean
  Constant : Constant  Value=VerboseSignal
  Subsystem : Subsystem
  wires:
  Constant/1 -> Compare To Constant/1
  Compare To Constant/1 -> Subsystem/Enable
  iner_kgm2/1 -> Subsystem/3(iner_kgm2)
  spd_radps/1 -> Subsystem/2(spd_radps)
  " trq_Nm"/1 -> Subsystem/1(" trq_Nm")

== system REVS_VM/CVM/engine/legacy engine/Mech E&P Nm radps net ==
  " trq_Nm" : Inport
  spd_radps : Inport  Port=2
  iner_kgm2 : Inport  Port=3
  Compare To Constant : simulink/Logic and Bit Operations/Compare To Constant  relop=>=  const=1  OutDataTypeStr=boolean
  Constant : Constant  Value=VerboseSignal
  Subsystem : Subsystem
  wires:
  Constant/1 -> Compare To Constant/1
  Compare To Constant/1 -> Subsystem/Enable
  iner_kgm2/1 -> Subsystem/3(iner_kgm2)
  spd_radps/1 -> Subsystem/2(spd_radps)
  " trq_Nm"/1 -> Subsystem/1(" trq_Nm")

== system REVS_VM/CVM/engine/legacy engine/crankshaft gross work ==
  torque_Nm : Inport
  speed_radps : Inport  Port=2
  upstream_iner_kgm2 : Inport  Port=3
  Derivative : Derivative  CoefficientInTFapproximation=1e6
  Gain : Gain  Gain=1/1000
  Integrator1 : Integrator  UpperSaturationLimit=Inf  LowerSaturationLimit=0  ZeroCross=off
  Integrator2 : Integrator  UpperSaturationLimit=Inf  LowerSaturationLimit=0  ZeroCross=off
  Phase To Workspace : ToWorkspace  VariableName=result__phase_crankshaft_gross_pos_work_kJ  SampleTime=-1
  Pos : Fcn  Expr=u(1)*(u(1) >= 0)
  Product : Product
  Product1 : Product
  Product2 : Product
  Subtract : Sum  Inputs=+-
  Total To Workspace : ToWorkspace  VariableName=result__total_crankshaft_gross_pos_work_kJ  SampleTime=-1
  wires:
  Product2/1 -> Pos/1
  Pos/1 -> Gain/1
  Gain/1 -> Integrator1/1, Product/2
  Product1/1 -> Subtract/2
  Derivative/1 -> Product1/1
  speed_radps/1 -> Derivative/1, Product2/2
  upstream_iner_kgm2/1 -> Product1/2
  Subtract/1 -> Product2/1
  Integrator2/1 -> Phase To Workspace/1
  [REVS_phase_flag] -> Product/1
  Product/1 -> Integrator2/1
  Integrator1/1 -> Total To Workspace/1
  torque_Nm/1 -> Subtract/1

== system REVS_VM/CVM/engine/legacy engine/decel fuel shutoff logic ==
  system_bus : Inport
  Constant : Constant  Value=engine.decel_fuel_shutoff_disabled
  Logical Operator : Logic  Operator=OR  AllPortsSameDT=off  OutDataTypeStr=boolean
  Logical Operator1 : Logic  Operator=NOT  AllPortsSameDT=off  OutDataTypeStr=boolean
  dynamic equation : Subsystem
  eng_decel_fuel_cut_disable : Outport
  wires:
  Logical Operator1/1 -> Logical Operator/2
  dynamic equation/1(out) -> Logical Operator1/1
  system_bus/1 -> dynamic equation/1(bus)
  Constant/1 -> Logical Operator/1
  Logical Operator/1 -> eng_decel_fuel_cut_disable/1

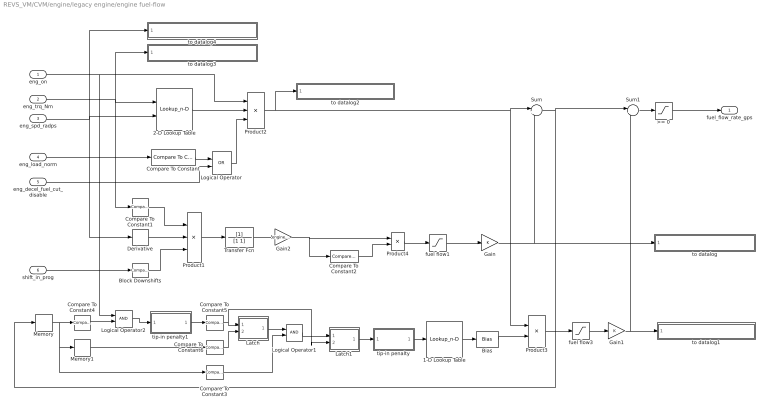
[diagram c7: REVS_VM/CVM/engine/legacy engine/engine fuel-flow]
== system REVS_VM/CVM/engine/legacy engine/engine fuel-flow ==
  eng_on : Inport
  eng_trq_Nm : Inport  Port=2
  eng_spd_radps : Inport  Port=3
  eng_load_norm : Inport  Port=4
  eng_decel_fuel_cut_disable : Inport  Port=5
  shift_in_prog : Inport  Port=6
  1-D Lookup Table : Lookup_n-D  NumberOfTableDimensions=1  BreakpointsForDimension1=engine.refuel_profile_time_secs  IndexSearchMethod=Linear search  BeginIndexSearchUsingPreviousIndexResult=on  Table=engine.refuel_profile_mult  ExtrapMethod=Clip  RndMeth=Simplest
  2-D Lookup Table : Lookup_n-D  BreakpointsForDimension1=engine.fuel_map_torque_Nm  BreakpointsForDimension2=engine.fuel_map_speed_radps  IndexSearchMethod=Linear search  BeginIndexSearchUsingPreviousIndexResult=on  Table=engine.fuel_map_gps  ExtrapMethod=Clip  UseLastTableValue=on  RndMeth=Simplest
  >= 0 : Saturate  UpperLimit=Inf  LowerLimit=0  ZeroCross=off
  Bias : Bias  Bias=-1
  Block Downshifts : simulink/Logic and Bit Operations/Compare To Constant  relop=>=  const=0  OutDataTypeStr=boolean  ZeroCross=off
  Compare To Constant : simulink/Logic and Bit Operations/Compare To Constant  relop=>=  const=0.001  OutDataTypeStr=boolean  ZeroCross=off
  Compare To Constant1 : simulink/Logic and Bit Operations/Compare To Constant  relop=>  const=0  OutDataTypeStr=boolean  ZeroCross=off
  Compare To Constant2 : simulink/Logic and Bit Operations/Compare To Constant  relop=>=  const=engine.acceleration_penalty_squelch_gps  OutDataTypeStr=boolean  ZeroCross=off
  Compare To Constant3 : simulink/Logic and Bit Operations/Compare To Constant  relop=~=  const=0  OutDataTypeStr=boolean  ZeroCross=off
  Compare To Constant4 : simulink/Logic and Bit Operations/Compare To Constant  relop=<=  const=0  OutDataTypeStr=boolean  ZeroCross=off
  Compare To Constant5 : simulink/Logic and Bit Operations/Compare To Constant  relop=>=  const=engine.refuel_min_defuel_duration_secs  OutDataTypeStr=boolean  ZeroCross=off
  Compare To Constant6 : simulink/Logic and Bit Operations/Compare To Constant  relop=~=  const=0  OutDataTypeStr=boolean  ZeroCross=off
  Derivative : Derivative
  Gain : Gain
  Gain1 : Gain
  Gain2 : Gain  Gain=engine.acceleration_penalty_gpradps2
  Latch : Subsystem
  Latch1 : Subsystem
  Logical Operator : Logic  Operator=OR  AllPortsSameDT=off  OutDataTypeStr=boolean
  Logical Operator1 : Logic  AllPortsSameDT=off  OutDataTypeStr=boolean
  Logical Operator2 : Logic  AllPortsSameDT=off  OutDataTypeStr=boolean
  Memory : Memory
  Memory1 : Memory
  Product1 : Product  Inputs=3
  Product2 : Product  Inputs=3
  Product3 : Product
  Product4 : Product
  Sum : Sum  Inputs=|++
  Sum1 : Sum  Inputs=|++
  Transfer Fcn : TransferFcn  Denominator=[1 1]
  fuel flow1 : Saturate  UpperLimit=inf  LowerLimit=0  ZeroCross=off
  fuel flow3 : Saturate  UpperLimit=engine.refuel_limit_gps  LowerLimit=0  ZeroCross=off
  tip-in penalty : Subsystem
  tip-in penalty1 : Subsystem
  to datalog : Subsystem
  to datalog1 : Subsystem
  to datalog2 : Subsystem
  to datalog3 : Subsystem
  to datalog4 : Subsystem
  fuel_flow_rate_gps : Outport
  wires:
  Logical Operator2/1 -> tip-in penalty1/1(bool)
  Compare To Constant2/1 -> Product4/2
  Gain2/1 -> Compare To Constant2/1, Product4/1
  Transfer Fcn/1 -> Gain2/1
  Product1/1 -> Transfer Fcn/1
  Derivative/1 -> Product1/2
  Product4/1 -> fuel flow1/1
  Block Downshifts/1 -> Product1/3
  shift_in_prog/1 -> Block Downshifts/1
  Sum/1 -> Memory/1, Sum1/1
  Bias/1 -> Product3/2
  fuel flow1/1 -> Gain/1
  Gain1/1 -> Sum1/2, to datalog1/1(Var)
  Gain/1 -> Sum/2, to datalog/1(Var)
  fuel flow3/1 -> Gain1/1
  Product3/1 -> fuel flow3/1
  Sum1/1 -> >= 0/1
  Latch1/1(State) -> tip-in penalty/1(bool)
  Logical Operator1/1 -> Latch1/1(On)
  Compare To Constant3/1 -> Logical Operator1/2
  Latch/1(State) -> Logical Operator1/1
  Memory1/1 -> Compare To Constant6/1
  Compare To Constant6/1 -> Latch/2(Off)
  Compare To Constant5/1 -> Latch/1(On), Latch1/2(Off)
  tip-in penalty1/1(out) -> Compare To Constant5/1
  Compare To Constant4/1 -> Logical Operator2/2
  Memory/1 -> Compare To Constant3/1, Memory1/1, Compare To Constant4/1
  1-D Lookup Table/1 -> Bias/1
  tip-in penalty/1(out) -> 1-D Lookup Table/1
  Compare To Constant1/1 -> Product1/1
  Product2/1 -> to datalog2/1(Var), Product3/1, Sum/1
  eng_trq_Nm/1 -> Compare To Constant1/1, to datalog3/1(Var), 2-D Lookup Table/1
  eng_spd_radps/1 -> 2-D Lookup Table/2, Derivative/1, to datalog4/1(Var)
  >= 0/1 -> fuel_flow_rate_gps/1
  Logical Operator/1 -> Product2/3
  Compare To Constant/1 -> Logical Operator/1
  2-D Lookup Table/1 -> Product2/2
  eng_on/1 -> Product2/1, Logical Operator2/1
  eng_load_norm/1 -> Compare To Constant/1
  eng_decel_fuel_cut_disable/1 -> Logical Operator/2

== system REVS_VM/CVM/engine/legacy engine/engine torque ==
  eng_slow_trq_Nm : Inport
  eng_fast_trq_Nm : Inport  Port=2
  eng_spd_radps : Inport  Port=3
  Boost Reponse : Subsystem
  Closed Throttle Torque Limit : Lookup_n-D  NumberOfTableDimensions=1  BreakpointsForDimension1=engine.closed_throttle_speed_radps  BeginIndexSearchUsingPreviousIndexResult=on  Table=engine.closed_throttle_torque_Nm  ExtrapMethod=Clip  UseLastTableValue=on  RndMeth=Simplest
  Full Throttle Torque Limit : Lookup_n-D  NumberOfTableDimensions=1  BreakpointsForDimension1=engine.full_throttle_speed_radps  BeginIndexSearchUsingPreviousIndexResult=on  Table=engine.full_throttle_torque_Nm  ExtrapMethod=Clip  UseLastTableValue=on  RndMeth=Simplest
  Gain : Gain  Gain=engine.fast_torque_fuel_adjust_norm
  Min1 : MinMax  Function=max  Inputs=2  ZeroCross=off
  Min2 : MinMax  Inputs=2  ZeroCross=off
  Min6 : MinMax  Inputs=2  ZeroCross=off
  Naturally Aspirated Torque Limit : Lookup_n-D  NumberOfTableDimensions=1  BreakpointsForDimension1=engine.naturally_aspirated_speed_radps  IndexSearchMethod=Linear search  BeginIndexSearchUsingPreviousIndexResult=on  Table=engine.naturally_aspirated_torque_Nm  ExtrapMethod=Clip  UseLastTableValue=on  RndMeth=Simplest
  Product : Product
  Product1 : Product  Inputs=*/
  Rate Limiter : RateLimiter  RisingSlewLimit=1/engine.throttle_duration_secs  FallingSlewLimit=-1/engine.throttle_duration_secs
  Sum1 : Sum
  Sum2 : Sum
  Sum3 : Sum  Inputs=+-
  Torque to Load (norm) : Subsystem
  eps : Saturate  UpperLimit=inf  LowerLimit=eps  ZeroCross=off
  reduce only : Saturate  UpperLimit=0  LowerLimit=-inf  ZeroCross=off
  to datalog1 : Subsystem
  to datalog2 : Subsystem
  to datalog3 : Subsystem
  to datalog4 : Subsystem
  to datalog5 : Subsystem
  to datalog6 : Subsystem
  to datalog7 : Subsystem
  eng_load_Nm : Outport
  eng_load_norm : Outport  Port=2
  eng_fuel_trq_Nm : Outport  Port=3
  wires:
  eps/1 -> Product1/2, Product/2
  Sum3/1 -> eps/1
  Boost Reponse/1(trq_limit_Nm) -> to datalog3/1(Var), Min6/1, Sum3/1
  Rate Limiter/1 -> Product/1
  Product1/1 -> Rate Limiter/1
  Min6/1 -> Product1/1
  Min2/1 -> Min1/1
  Min1/1 -> Torque to Load (norm)/1(torque), to datalog1/1(Var), eng_load_Nm/1
  eng_spd_radps/1 -> Full Throttle Torque Limit/1, Naturally Aspirated Torque Limit/1, Closed Throttle Torque Limit/1
  eng_fast_trq_Nm/1 -> to datalog6/1(Var), reduce only/1
  reduce only/1 -> Sum1/1, Gain/1
  Sum1/1 -> Min2/1
  Sum2/1 -> to datalog4/1(Var), eng_fuel_trq_Nm/1
  Gain/1 -> Sum2/1
  Product/1 -> Sum2/2, Sum1/2
  eng_slow_trq_Nm/1 -> Boost Reponse/1(target_trq_Nm), to datalog5/1(Var), Min6/2
  Naturally Aspirated Torque Limit/1 -> to datalog7/1(Var), Boost Reponse/3(nat_asp_trq_Nm)
  Full Throttle Torque Limit/1 -> Boost Reponse/2(max_trq_Nm), Min2/2, Torque to Load (norm)/2(max)
  Closed Throttle Torque Limit/1 -> Sum3/2, Min1/2, Torque to Load (norm)/3(min)
  Torque to Load (norm)/1(load_norm) -> to datalog2/1(Var), eng_load_norm/1

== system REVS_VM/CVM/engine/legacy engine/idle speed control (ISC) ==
  system_bus : Inport
  eng_spd_radps : Inport  Port=2
  eng_min_trq_Nm : Inport  Port=3
  " Sat >= 0" : Saturate  UpperLimit=inf  LowerLimit=0  ZeroCross=off
  Add : Sum  Inputs=+++-+
  Derivative : Derivative
  Derivative1 : Derivative
  Derivative2 : Derivative
  ISC state : Subsystem
  Integrator : Integrator  ExternalReset=level  LimitOutput=on  UpperSaturationLimit=Inf  LowerSaturationLimit=0
  Kd : Gain  Gain=engine.idle_control_Kd
  Ki : Gain  Gain=engine.idle_control_Ki
  Kp : Gain  Gain=engine.idle_control_Kp
  Logical Operator : Logic  Operator=NOT  AllPortsSameDT=off  OutDataTypeStr=boolean
  Product3 : Product
  Subsystem : Subsystem
  Sum1 : Sum  Inputs=+-
  Sum2 : Sum  Inputs=-+
  driver bus1 : BusSelector  OutputSignals=powertrain.control.ctrl_eng_on,powertrain.trans.ctrl.eng_des_spd_radps
  eng iner : Gain  Gain=engine.inertia_kgm2
  eng iner2 : Gain  Gain=engine.inertia_kgm2 * 2
  gain : Gain  Gain=0.9
  sat >= 0 : Saturate  UpperLimit=Inf  LowerLimit=0  ZeroCross=off
  to datalog1 : Subsystem
  to datalog2 : Subsystem
  to datalog3 : Subsystem
  to datalog4 : Subsystem
  to datalog5 : Subsystem
  to datalog6 : Subsystem
  trq_out_Nm : Outport
  target_idle_spd_radps : Outport  Port=2
  ISC_state : Outport  Port=3
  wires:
  eng iner2/1 -> Add/5, to datalog4/1(Var)
  gain/1 -> Add/4
  Kp/1 -> Add/1, to datalog3/1(Var)
  eng_min_trq_Nm/1 -> gain/1
  Sum1/1 -> eng iner2/1
  Derivative2/1 -> Sum1/1
  Derivative1/1 -> Sum1/2
  Sum2/1 -> eng iner/1
  sat >= 0/1 -> Derivative/1
  ISC state/1(state) -> Logical Operator/1, ISC_state/1, Product3/1, Subsystem/4(ISC_state), to datalog6/1(Var)
  driver bus1/2 -> Subsystem/2(eng_des_spd_radps)  "<eng_des_spd_radps>"
  Subsystem/1(target_idle_spd_radps) -> to datalog5/1(Var), Derivative2/1, target_idle_spd_radps/1, Sum2/2
  eng iner/1 -> Ki/1, Kd/1, Kp/1
  Integrator/1 -> Add/2, to datalog2/1(Var)
  " Sat >= 0"/1 -> trq_out_Nm/1, to datalog1/1(Var)
  eng_spd_radps/1 -> ISC state/2(eng_spd_radps), Sum2/1, Subsystem/3(eng_spd_radps), Derivative1/1
  Derivative/1 -> Add/3
  Ki/1 -> Integrator/1
  Add/1 -> Product3/2
  Kd/1 -> sat >= 0/1
  Product3/1 -> " Sat >= 0"/1
  Logical Operator/1 -> Integrator/2
  system_bus/1 -> driver bus1/1, Subsystem/1(system_bus)
  driver bus1/1 -> ISC state/1(eng_on)  "<ctrl_eng_on>"

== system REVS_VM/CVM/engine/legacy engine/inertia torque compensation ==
  eng_on : Inport
  comp_iner_enable : Inport  Port=2
  eng_spd_radps : Inport  Port=3
  iner_kgm2 : Inport  Port=4
  load_norm : Inport  Port=5
  <= 0 : Saturate  UpperLimit=0  LowerLimit=-Inf  ZeroCross=off
  Memory : Memory
  Product : Product  Inputs=5
  Transfer Fcn : TransferFcn  Numerator=[1 0]  Denominator=[0.02 1]
  downstream compensation : Gain  Gain=1.5
  load based inertia adj. norm : Lookup_n-D  NumberOfTableDimensions=1  BreakpointsForDimension1=[0, 0.65, 0.90, 1.0]  Table=[1.0, 1.0, 0.0, 0.0]  InternalRulePriority=Speed  RndMeth=Simplest
  to datalog1 : Subsystem
  comp_trq_Nm : Outport
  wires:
  Product/1 -> <= 0/1
  load based inertia adj. norm/1 -> Product/5
  Memory/1 -> load based inertia adj. norm/1
  load_norm/1 -> Memory/1
  eng_on/1 -> Product/1
  <= 0/1 -> comp_trq_Nm/1, to datalog1/1(Var)
  iner_kgm2/1 -> downstream compensation/1
  eng_spd_radps/1 -> Transfer Fcn/1
  Transfer Fcn/1 -> Product/3
  downstream compensation/1 -> Product/4
  comp_iner_enable/1 -> Product/2
